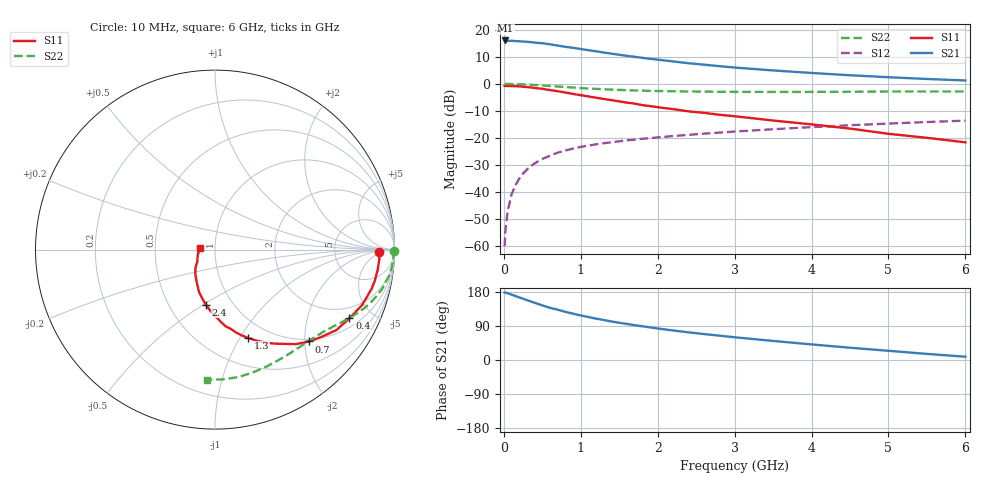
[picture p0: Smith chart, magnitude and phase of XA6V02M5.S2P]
! SIEMENS Discrete & RF Semiconductors
! BFY180
! Si NPN RF Bipolar Junction Transistor in MICRO-X
! VCE = 6 V  IC = 2.5 mA
! Common Emitter S-Parameters:  May  1997
# GHz  S  MA  R  50
!  f  S11  S21  S12  S22
! GHz  MAG  ANG  MAG  ANG  MAG  ANG  MAG  ANG
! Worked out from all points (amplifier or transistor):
!   36 points, 10 MHz to 6 GHz, reference 50 ohm
!   highest |S21| = 16.1 dB at 20 MHz (marker M1)
!   |S21| within 3 dB of that: start of sweep to 964.6 MHz
!   unconditionally stable (mu >= 1): 2.771 GHz to end of sweep
!   at 250 MHz: K = 0.14, MSG = 24.4 dB, |S12| = -33.1 dB
!   at 1.4 GHz: K = 0.71, MSG = 16.4 dB, |S12| = -21.6 dB
!   at 6 GHz: K = 1.06, MAG = 6.0 dB, |S12| = -13.6 dB
!   S11 on the Smith chart (normalised r, x): 10 MHz: 22, -3; 400 MHz: 1.40, -3.65; 700 MHz: 0.95, -2.10; 1.3 GHz: 0.80, -1.09; 2.4 GHz: 0.75, -0.51; 6 GHz: 0.85, +0.02
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0.01  0.9159 -0.7  6.313 178.3  0.001 79.3  0.9947 -0.3
0.02  0.9156 -1.3  6.355 177.7  0.0019 91.1  0.9997 -0.7
0.05  0.917 -3.4  6.214 176.2  0.0045 88.0  0.9956 -1.7
0.1  0.9134 -7.1  6.275 172.6  0.009 86.7  0.9932 -3.6
0.15  0.9074 -10.9  6.186 168.9  0.0133 84.5  0.9911 -5.3
0.3  0.8756 -20.7  6.007 157.9  0.0261 78.0  0.9709 -10.3
0.4  0.8408 -27.1  5.804 151.0  0.034 73.4  0.9559 -13.3
0.5  0.8118 -33.5  5.642 144.1  0.0409 70.0  0.9357 -16.2
0.6  0.7674 -39.3  5.394 137.6  0.0472 66.5  0.9156 -18.8
0.7  0.7331 -44.3  5.111 132.8  0.0536 63.8  0.8948 -21.3
0.9  0.6511 -53.8  4.647 122.3  0.0639 58.8  0.8569 -25.3
1.1  0.5863 -61.9  4.191 113.4  0.0723 55.4  0.8222 -28.8
1.3  0.5262 -69.4  3.795 105.5  0.0801 52.3  0.7951 -31.9
1.5  0.4748 -75.9  3.458 98.2  0.087 50.2  0.7735 -34.8
1.7  0.432 -82.0  3.171 91.9  0.0932 48.2  0.7562 -37.4
2.2  0.3418 -94.3  2.603 78.0  0.1087 44.3  0.7316 -43.9
2.4  0.311 -99.5  2.41 73.0  0.1142 42.9  0.7233 -46.4
3  0.2525 -110.6  2.006 60.0  0.1315 38.8  0.7135 -53.7
3.5  0.2103 -118.8  1.774 50.3  0.1452 35.7  0.7104 -59.8
4.5  0.1492 -136.9  1.445 32.4  0.172 28.6  0.7161 -72.7
5.5  0.1007 -162.8  1.233 16.1  0.1973 21.0  0.7247 -86.6
6  0.0832 173.7  1.157 8.6  0.2091 16.8  0.7256 -93.5
